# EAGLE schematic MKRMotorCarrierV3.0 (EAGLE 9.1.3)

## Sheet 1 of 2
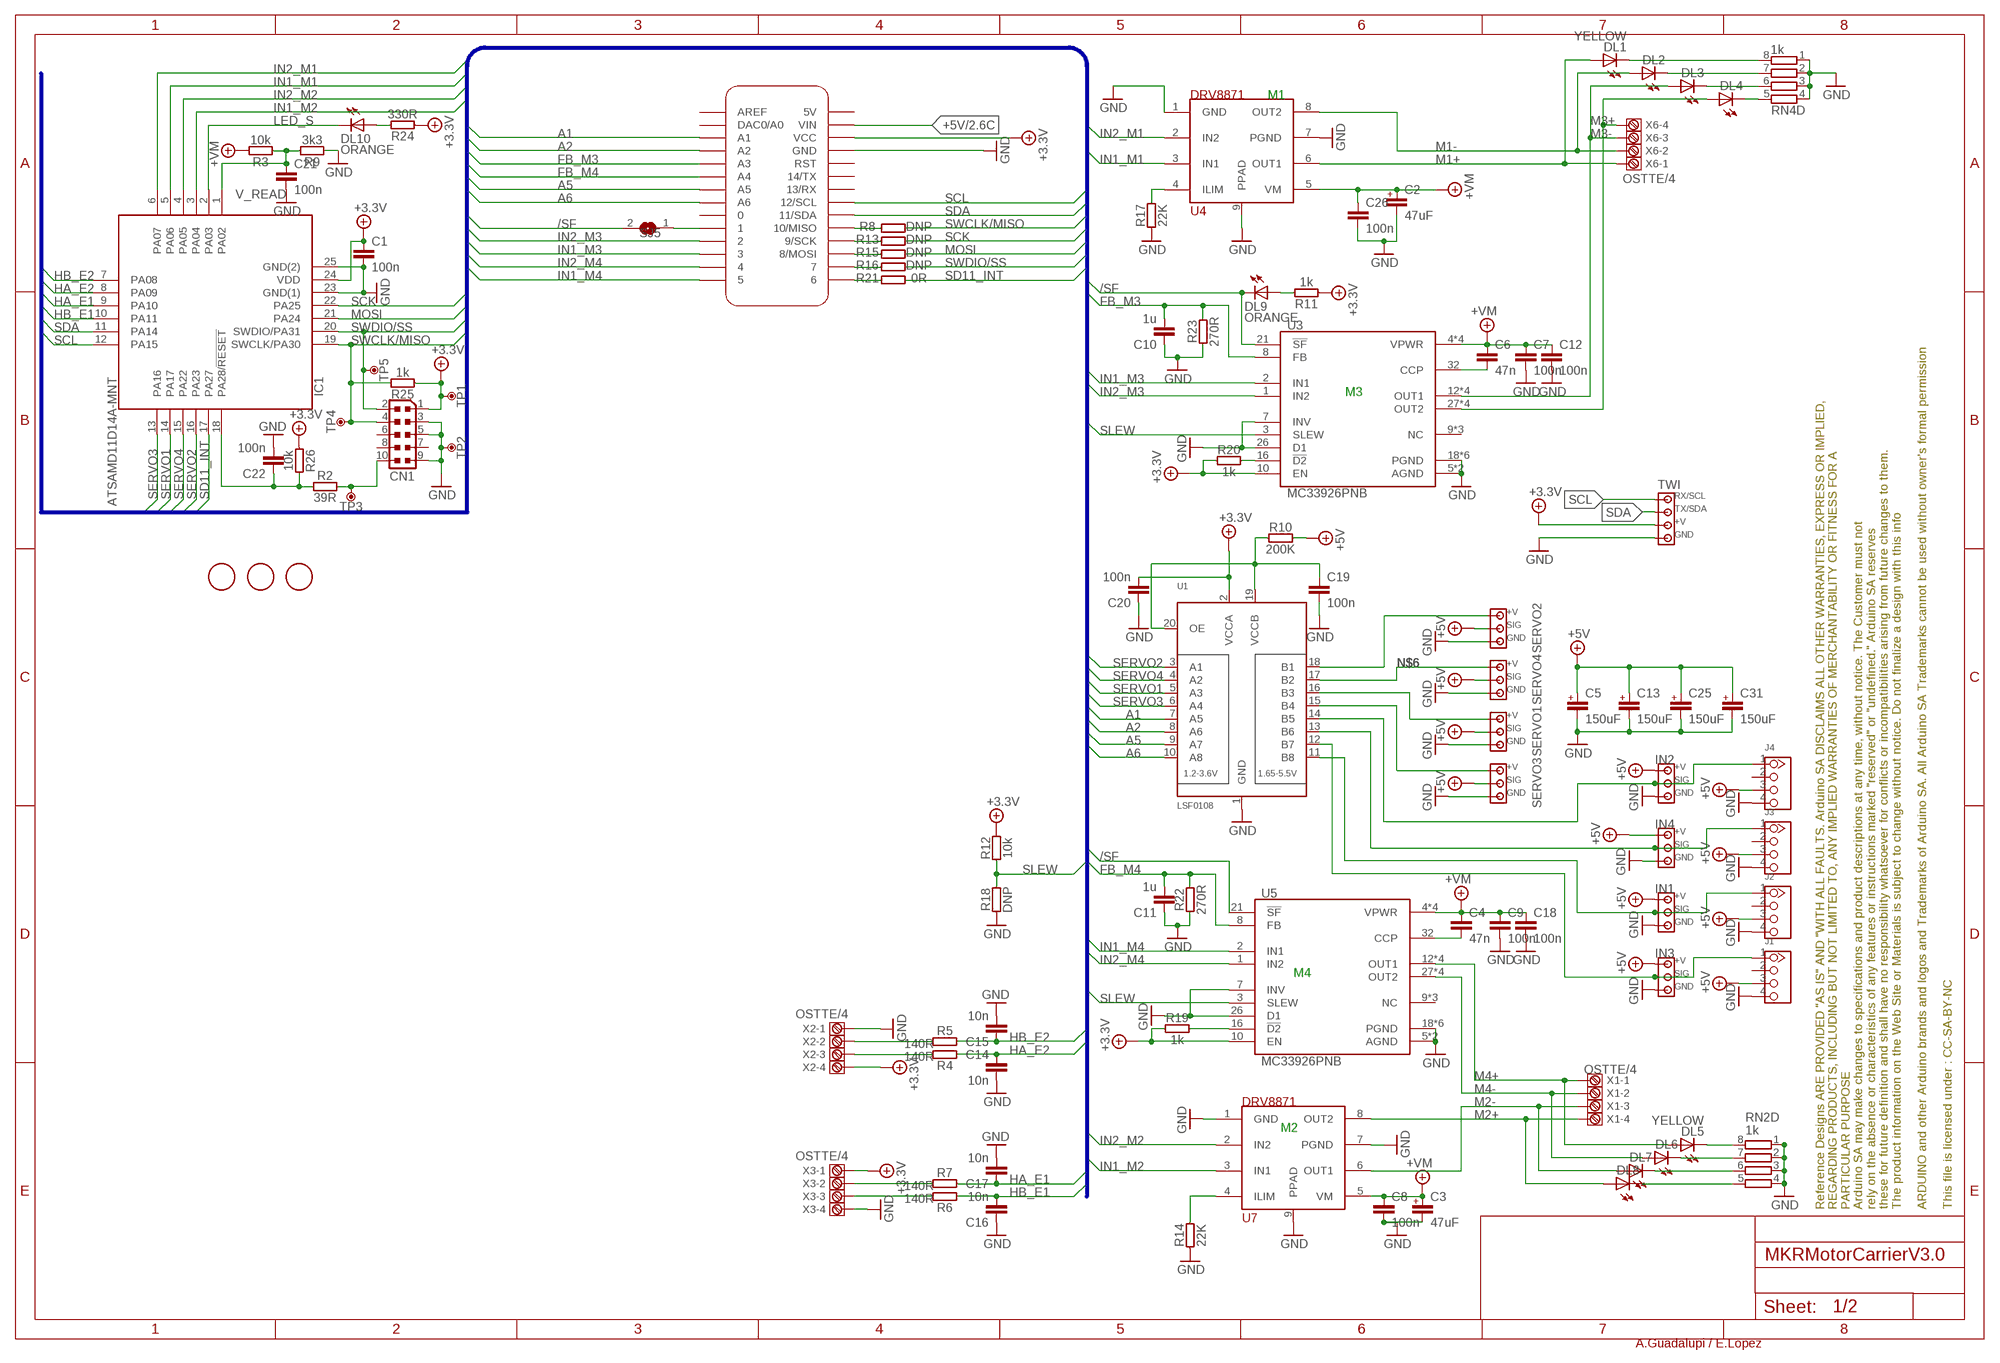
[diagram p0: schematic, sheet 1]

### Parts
C1  100n  C-100NF-0402  [0402-1005X55N]
C2  47uF  C+-47UFAVX-TCJ  [SMC_B]
C3  47uF  C+-47UFAVX-TCJ  [SMC_B]
C4  47n  C-47N-0402  [0402-1005X55N]
C5  150uF  C+PAN-C  [PANASONIC_C]
C6  47n  C-47N-0402  [0402-1005X55N]
C7  100n  C-100NF-0402  [0402-1005X55N]
C8  100n  C-100NF-0402  [0402-1005X55N]
C9  100n  C-100NF-0402  [0402-1005X55N]
C10  1u  C-1UF-0402  [0402-1005X55N]
C11  1u  C-1UF-0402  [0402-1005X55N]
C12  100n  C-100NF-0402  [0402-1005X55N]
C13  150uF  C+PAN-C  [PANASONIC_C]
C14  10n  C-10NF-0402  [0402-1005X55N]
C15  10n  C-10NF-0402  [0402-1005X55N]
C16  10n  C-10NF-0402  [0402-1005X55N]
C17  10n  C-10NF-0402  [0402-1005X55N]
C18  100n  C-100NF-0402  [0402-1005X55N]
C19  100n  C-100NF-0402  [0402-1005X55N]
C20  100n  C-100NF-0402  [0402-1005X55N]
C21  100n  C-100NF-0402  [0402-1005X55N]
C22  100n  C-100NF-0402  [0402-1005X55N]
C25  150uF  C+PAN-C  [PANASONIC_C]
C26  100n  C-100NF-0402  [0402-1005X55N]
C31  150uF  C+PAN-C  [PANASONIC_C]
CN1  DNP  JTAG_CONNECTOR-ROUND  [PINHEAD_2X05_127]
DL1  YELLOW  LED-YELLOW-0603  [LEDC1608X80N-AK]
DL2  YELLOW  LED-YELLOW-0603  [LEDC1608X80N-AK]
DL3  YELLOW  LED-YELLOW-0603  [LEDC1608X80N-AK]
DL4  YELLOW  LED-YELLOW-0603  [LEDC1608X80N-AK]
DL5  YELLOW  LED-YELLOW-0603  [LEDC1608X80N-AK]
DL6  YELLOW  LED-YELLOW-0603  [LEDC1608X80N-AK]
DL7  YELLOW  LED-YELLOW-0603  [LEDC1608X80N-AK]
DL8  YELLOW  LED-YELLOW-0603  [LEDC1608X80N-AK]
DL9  ORANGE  LED-ORANGE-0603  [LEDC1608X80N-AK]
DL10  ORANGE  LED-ORANGE-0603  [LEDC1608X80N-AK]
FRAME2  DNP  A3-FRAME-STANDARD  [FRAME]
IC1  ATSAMD11D14A-MNT  [QFN50P400X400X90-25N]
IN1  DNP  MODULINO-3-DNPSM  [MODULINO-3SM]
IN2  DNP  MODULINO-3-DNPSM  [MODULINO-3SM]
IN3  DNP  MODULINO-3-DNPSM  [MODULINO-3SM]
IN4  DNP  MODULINO-3-DNPSM  [MODULINO-3SM]
J1  DNP  GROVE-CONNECTOR-DNP  [HW4-2.0]
J2  DNP  GROVE-CONNECTOR-DNP  [HW4-2.0]
J3  DNP  GROVE-CONNECTOR-DNP  [HW4-2.0]
J4  DNP  GROVE-CONNECTOR-DNP  [HW4-2.0]
R2  39R  R-39R-0402  [0402-1005X55N]
R3  10k  R-10K-0402  [0402-1005X55N]
R4  140R  R-140R-0402  [0402-1005X55N]
R5  140R  R-140R-0402  [0402-1005X55N]
R6  140R  R-140R-0402  [0402-1005X55N]
R7  140R  R-140R-0402  [0402-1005X55N]
R8  DNP  R-DNP-0402  [0402-1005X55N]
R9  3k3  R-3K3-0402  [0402-1005X55N]
R10  200K  R-200K-0402  [0402-1005X55N]
R11  1k  R-1K-0402  [0402-1005X55N]
R12  10k  R-10K-0402  [0402-1005X55N]
R13  DNP  R-DNP-0402  [0402-1005X55N]
R14  22K  R-22K-0402  [0402-1005X55N]
R15  DNP  R-DNP-0402  [0402-1005X55N]
R16  DNP  R-DNP-0402  [0402-1005X55N]
R17  22K  R-22K-0402  [0402-1005X55N]
R18  DNP  R-DNP-0402  [0402-1005X55N]
R19  1k  R-1K-0402  [0402-1005X55N]
R20  1k  R-1K-0402  [0402-1005X55N]
R21  0R  R-0R-0402  [0402-1005X55N]
R22  270R  R-270R-0402  [0402-1005X55N]
R23  270R  R-270R-0402  [0402-1005X55N]
R24  330R  R-330R-0402  [0402-1005X55N]
R25  1k  R-1K-0402  [0402-1005X55N]
R26  10k  R-10K-0402  [0402-1005X55N]
RN2  1k  4R-N-1KCAY16  [CAY16]
RN4  1k  4R-N-1KCAY16  [CAY16]
SERVO1  DNP  MODULINO-3-DNPSM  [MODULINO-3SM]
SERVO2  DNP  MODULINO-3-DNPSM  [MODULINO-3SM]
SERVO3  DNP  MODULINO-3-DNPSM  [MODULINO-3SM]
SERVO4  DNP  MODULINO-3-DNPSM  [MODULINO-3SM]
SJ5  SJ  [SJ]
TP1  DNP  TPTP-1.00MM  [TP-1.00MM]
TP2  DNP  TPTP-1.00MM  [TP-1.00MM]
TP3  DNP  TPTP-1.00MM  [TP-1.00MM]
TP4  DNP  TPTP-1.00MM  [TP-1.00MM]
TP5  DNP  TPTP-1.00MM  [TP-1.00MM]
TWI  -  MODULINO-4  [MODULINO-4]
U1  LSF0108  LSF0108PWR  [TSSOP20]
U3  MC33926PNB  [32-PQFN(8X8)]
U4  DRV8871  [SOIC127P600X170-8N]
U5  MC33926PNB  [32-PQFN(8X8)]
U7  DRV8871  [SOIC127P600X170-8N]
U$1  MKRBOARD4CARRIER  [MKRBOARD-4CARRIER]
U$33  DNP  FIDUCIAL-1.5MM  [FD-1-1.5]
U$34  DNP  FIDUCIAL-1.5MM  [FD-1-1.5]
U$35  DNP  FIDUCIAL-1.5MM  [FD-1-1.5]
X1  OSTTE/4  [OSTTE/4]
X2  OSTTE/4  [OSTTE/4]
X3  OSTTE/4  [OSTTE/4]
X6  OSTTE/4  [OSTTE/4]

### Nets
+3.3V: C1.1 C20.2 CN1.1 IC1.24(VDD) R11.1 R12.2 R19.1 R20.1 R24.1 R25.1 R26.1 TP1.X TWI.3 U1.2(VCCA) U3.10(EN) U5.10(EN) U$1.VCC X2.4 X3.1 ; also sheet 2
+5V: C5.+ C13.+ C25.+ C31.+ IN1.1 IN2.1 IN3.1 IN4.1 J1.3 J2.3 J3.3 J4.3 R10.2 SERVO1.2 SERVO2.2 SERVO3.2 SERVO4.2 U$1.VIN ; also sheet 2
+VM: C2.+ C3.+ C4.1 C6.1 C7.1 C8.1 C9.1 C12.1 C18.1 C26.1 R3.2 U3.4(VPWR) U3.6(VPWR) U3.11(VPWR) U3.31(VPWR) U4.5(VM) U5.4(VPWR) U5.6(VPWR) U5.11(VPWR) U5.31(VPWR) U7.5(VM) ; also sheet 2
/SF: DL9.C SJ5.2 U3.21(!SF) U5.21(!SF)
A1: U1.7(A5) U$1.A1
A2: U1.8(A6) U$1.A2
A5: U1.9(A7) U$1.A5
A6: U1.10(A8) U$1.A6
FB_M3: C10.2 R23.2 U3.8(FB) U$1.A3
FB_M4: C11.2 R22.2 U5.8(FB) U$1.A4
GND: C1.2 C2.- C3.- C5.- C7.2 C8.2 C9.2 C10.1 C11.1 C12.2 C13.- C14.1 C15.2 C16.1 C17.2 C18.2 C19.2 C20.1 C21.2 C22.2 C25.- C26.2 C31.- CN1.3 CN1.5 CN1.9 IC1.23(GND(1)) IC1.25(GND(2)) IN1.3 IN2.3 IN3.3 IN4.3 J1.4 J2.4 J3.4 J4.4 R9.1 R14.1 R17.1 R18.1 R22.1 R23.1 RN2.1 RN2.2 RN2.3 RN2.4 RN4.1 RN4.2 RN4.3 RN4.4 SERVO1.3 SERVO2.3 SERVO3.3 SERVO4.3 TP2.X TWI.4 U1.1(GND) U3.5(AGND) U3.7(INV) U3.18(PGND) U3.19(PGND) U3.20(PGND) U3.22(PGND) U3.23(PGND) U3.24(PGND) U3.26(D1) U3.EPAD(AGND) U4.1(GND) U4.7(PGND) U4.9(PPAD) U5.5(AGND) U5.7(INV) U5.18(PGND) U5.19(PGND) U5.20(PGND) U5.22(PGND) U5.23(PGND) U5.24(PGND) U5.26(D1) U5.EPAD(AGND) U7.1(GND) U7.7(PGND) U7.9(PPAD) U$1.GND X2.1 X3.4 ; also sheet 2
HA_E1: C17.1 IC1.9(PA10) R7.1
HA_E2: C14.2 IC1.8(PA09) R4.1
HB_E1: C16.2 IC1.10(PA11) R6.1
HB_E2: C15.1 IC1.7(PA08) R5.1
IN1_A6: IN1.2 J2.1 U1.11(B8)
IN1_M1: IC1.5(PA06) U4.3(IN1)
IN1_M2: IC1.3(PA04) U7.3(IN1)
IN1_M3: U3.2(IN1) U$1.3
IN1_M4: U5.2(IN1) U$1.5
IN2_A1: IN2.2 J4.1 U1.14(B5)
IN2_M1: IC1.6(PA07) U4.2(IN2)
IN2_M2: IC1.4(PA05) U7.2(IN2)
IN2_M3: U3.1(IN2) U$1.2
IN2_M4: U5.1(IN2) U$1.4
IN3_A5: IN3.2 J1.1 U1.12(B7)
IN4_A2: IN4.2 J3.1 U1.13(B6)
LED_S: DL10.C IC1.2(PA03)
M1+: DL1.A U4.6(OUT1) X6.1
M1-: DL2.A U4.8(OUT2) X6.2
M2+: DL8.A U7.8(OUT2) X1.4
M2-: DL7.A U7.6(OUT1) X1.3
M3+: DL4.A U3.27(OUT2) U3.28(OUT2) U3.29(OUT2) U3.30(OUT2) X6.4
M3-: DL3.A U3.12(OUT1) U3.13(OUT1) U3.14(OUT1) U3.15(OUT1) X6.3
M4+: DL5.A U5.12(OUT1) U5.13(OUT1) U5.14(OUT1) U5.15(OUT1) X1.1
M4-: DL6.A U5.27(OUT2) U5.28(OUT2) U5.29(OUT2) U5.30(OUT2) X1.2
MOSI: IC1.21(PA24) R15.1
N$2: R6.2 X3.3
N$4: SERVO1.1 U1.16(B3)
N$6: SERVO4.1 U1.17(B2)
N$7: SERVO2.1 U1.18(B1)
N$9: SERVO3.1 U1.15(B4)
N$10: R7.2 X3.2
N$11: R5.2 X2.2
N$12: R4.2 X2.3
N$13: DL9.A R11.2
N$14: CN1.10 R2.2 TP3.X
N$15: C22.1 IC1.18(PA28/!RESET) R2.1 R26.2
N$16: SJ5.1 U$1.1
N$17: DL1.C RN4.8
N$18: C19.1 R10.1 U1.19(VCCB) U1.20(OE)
N$20: DL2.C RN4.7
N$21: DL3.C RN4.6
N$24: DL5.C RN2.8
N$25: DL4.C RN4.5
N$26: DL6.C RN2.7
N$28: C6.2 U3.32(CCP)
N$30: C4.2 U5.32(CCP)
N$31: DL7.C RN2.6
N$32: DL8.C RN2.5
N$35: R20.2 U3.16(!D2)
N$36: R17.2 U4.4(ILIM)
N$37: R19.2 U5.16(!D2)
N$38: R21.1 U$1.6
N$39: R14.2 U7.4(ILIM)
N$40: R8.2 U$1.10(10/MISO)
N$41: R13.2 U$1.9(9/SCK)
N$42: DL10.A R24.2
N$43: R15.2 U$1.8(8/MOSI)
N$45: R16.2 U$1.7
SCK: IC1.22(PA25) R13.1
SCL: IC1.12(PA15) TWI.1 U$1.12(12/SCL)
SD11_INT: IC1.17(PA27) R21.2
SDA: IC1.11(PA14) TWI.2 U$1.11(11/SDA)
SERVO1: IC1.14(PA17) U1.5(A3)
SERVO2: IC1.16(PA23) U1.3(A1)
SERVO3: IC1.13(PA16) U1.6(A4)
SERVO4: IC1.15(PA22) U1.4(A2)
SLEW: R12.1 R18.2 U3.3(SLEW) U5.3(SLEW)
SWCLK/MISO: CN1.4 IC1.19(SWCLK/PA30) R8.1 R25.2 TP4.X
SWDIO/SS: CN1.2 IC1.20(SWDIO/PA31) R16.1 TP5.X
V_READ: C21.1 IC1.1(PA02) R3.1 R9.2
Unconnected: CN1.6 CN1.7 CN1.8 J1.2 J2.2 J3.2 J4.2 U3.9(NC) U3.17(NC) U3.25(NC) U5.9(NC) U5.17(NC) U5.25(NC) U$1.0 U$1.5V U$1.13(13/RX) U$1.14(14/TX) U$1.A0(DAC0/A0) U$1.AREF U$1.RST

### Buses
MOSI,MISO,SCK,SS,SDA,SCL,A1,A2,A4,A3,A6,A5,FB_M3,FB_M4,IN1_M3,IN1_M4,IN1_M1,IN1_M2,IN2_M1,IN2_M2,IN2_M3,IN2_M4,SERVO1,SERVO2,SERVO3,SERVO4,HA_E1,HA_E2,HB_E1,HB_E2,VIN,/SF,SLEW,SD11_INT,SWDIO/SS,SWCLK/MISO

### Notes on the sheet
- M1
- M3
- M4
- M2
- A.Guadalupi / E.Lopez

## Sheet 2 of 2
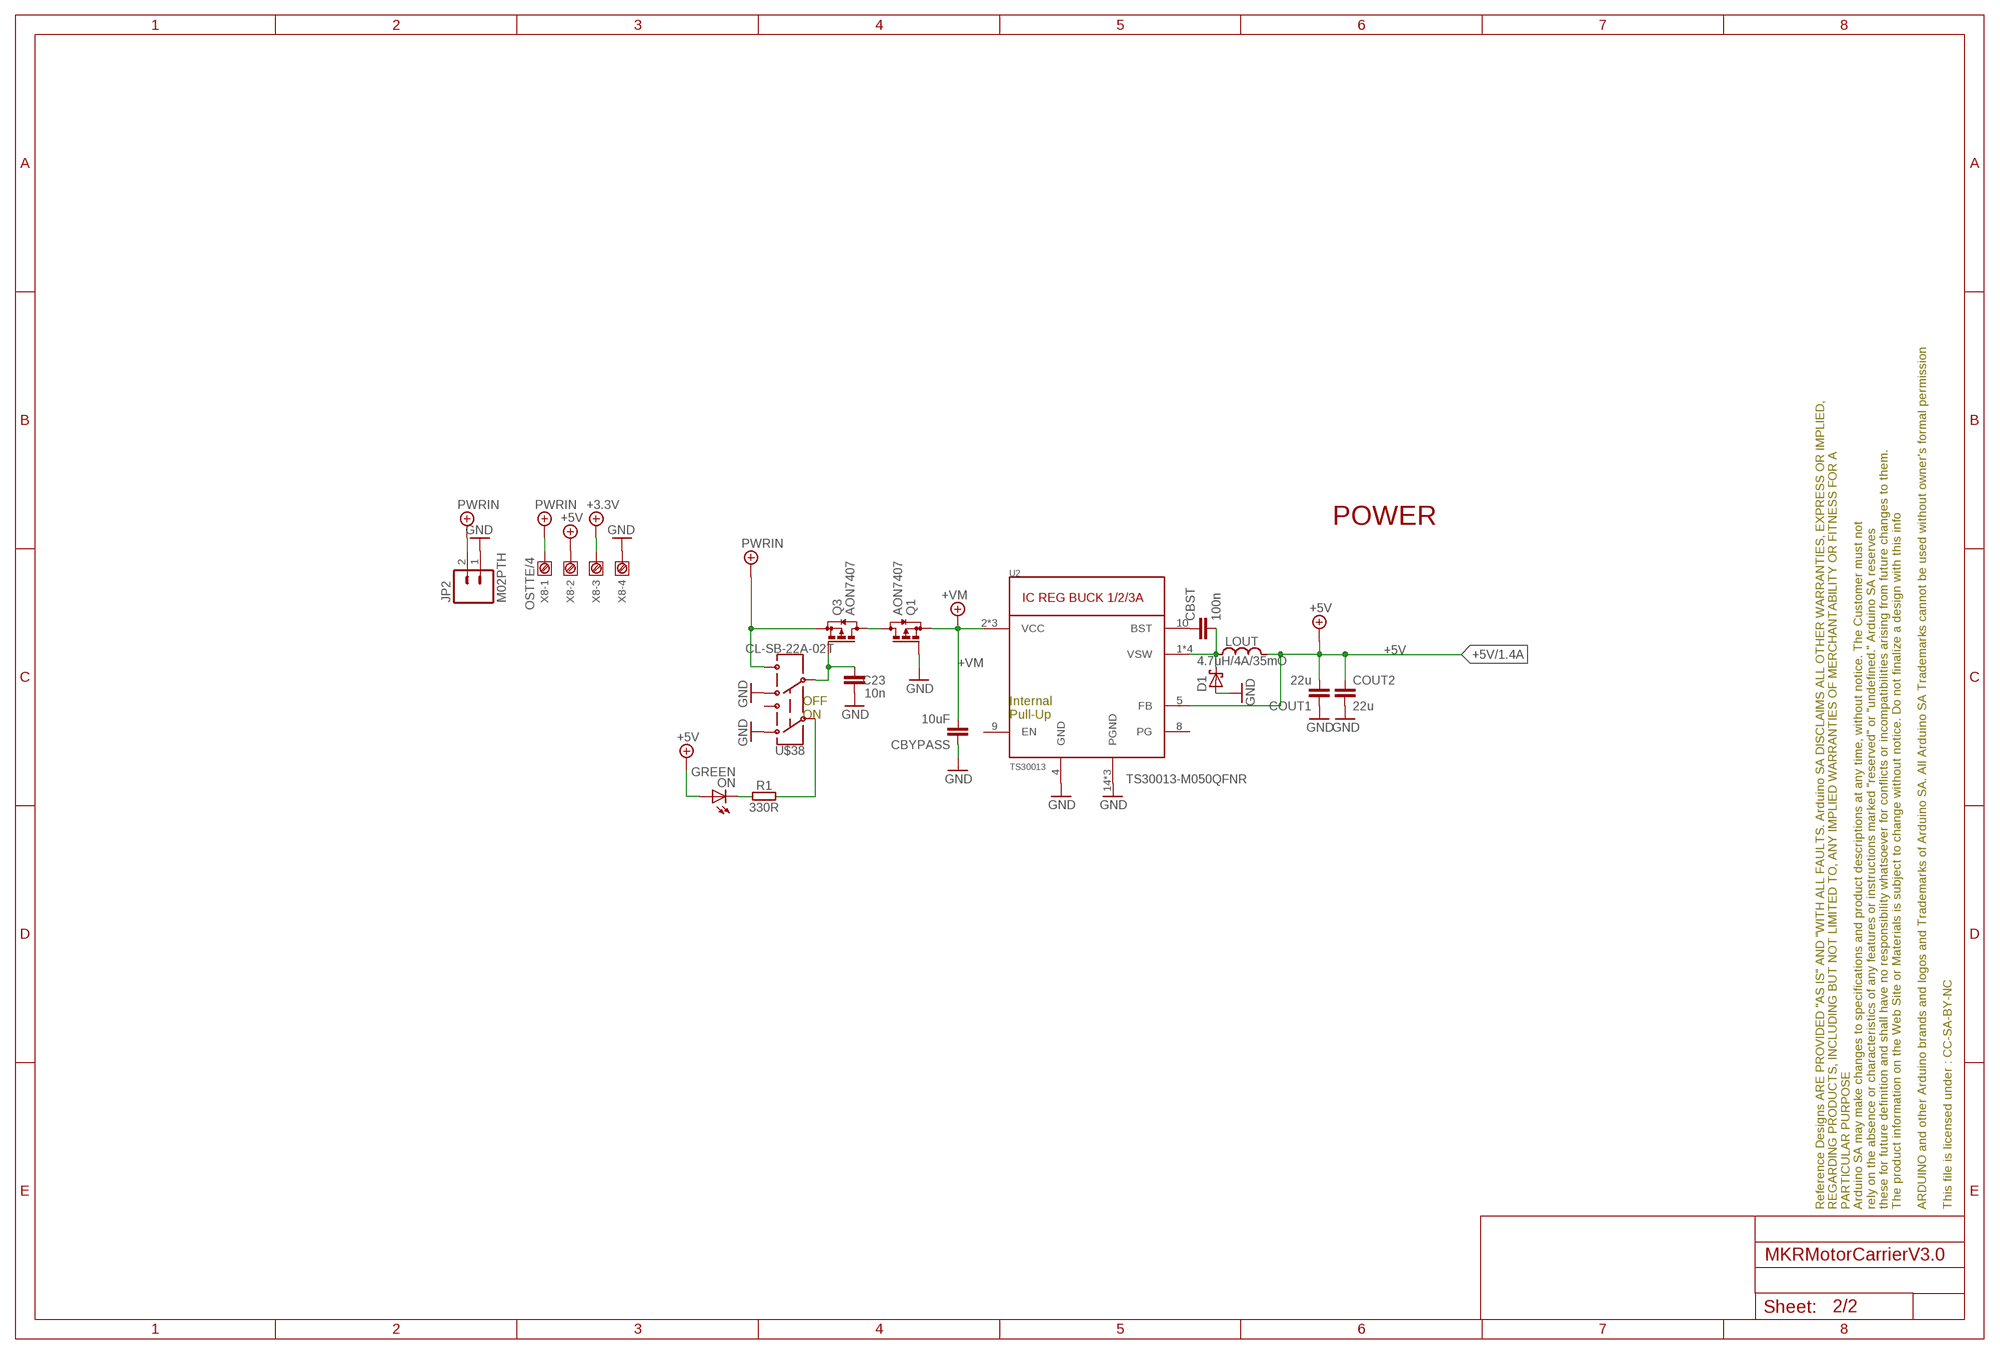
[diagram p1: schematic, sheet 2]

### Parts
C23  10n  C-10NF-0402  [0402-1005X55N]
CBST  100n  C-100NF-0402  [0402-1005X55N]
CBYPASS  10uF  C-10UF-1206  [C1206]
COUT1  22u  C-22U-0805  [0805-R2013X50N]
COUT2  22u  C-22U-0805  [0805-R2013X50N]
D1  40V/5A  D_SCHOTTKY-PMEG4050EP  [SOD-128]
FRAME1  DNP  A3-FRAME-NO-BAN  [FRAME-NO-BAN]
JP2  M02PTH  [1X02]
LOUT  4.7uH/4A/35mO  LVLS6045EX-4R7M  [6X6_NON-STANDARD]
ON  GREEN  LED-GREEN-0603  [LEDC1608X80N-AK]
Q1  AON7407  [DFN3X3_8L]
Q3  AON7407  [DFN3X3_8L]
R1  330R  R-330R-0402  [0402-1005X55N]
U2  TS30013  TS3001XTS30013  [QFN16]
U$38  CL-SB-22A-02T  [CL-SB-22A]
X8  OSTTE/4  [OSTTE/4]

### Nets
+3.3V: X8.3 ; also sheet 1
+5V: COUT1.2 COUT2.1 LOUT.P$2 ON.A U2.5(FB) X8.2 ; also sheet 1
+VM: CBYPASS.2 Q1.P$1(S) Q1.P$2(S) Q1.P$3(S) U2.2(VCC) U2.3(VCC) U2.11(VCC) ; also sheet 1
GND: C23.1 CBYPASS.1 COUT1.1 COUT2.2 D1.P$2(A) JP2.1 Q1.P$4(G) U2.4(GND) U2.14(PGND) U2.15(PGND) U2.17(PGND) U$38.P$1 U$38.P$4 X8.4 ; also sheet 1
N$3: CBST.1 U2.10(BST)
N$5: CBST.2 D1.P$1(C) LOUT.P$1 U2.1(VSW) U2.12(VSW) U2.13(VSW) U2.16(VSW)
N$19: R1.2 U$38.P$2
N$22: Q1.P$5(D) Q1.P$6(D) Q1.P$7(D) Q3.P$5(D) Q3.P$6(D) Q3.P$7(D)
N$23: C23.2 Q3.P$4(G) U$38.P$5
N$133: ON.C R1.1
PWRIN: JP2.2 Q3.P$1(S) Q3.P$2(S) Q3.P$3(S) U$38.P$6 X8.1
Unconnected: U2.8(PG) U2.9(EN) U$38.P$3

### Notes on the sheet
- POWER
- OFF
  ON
- Internal
  Pull-Up
- TS30013-M050QFNR

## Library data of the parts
C1 C7-C9 C12 C18-C22 C26 CBST = Arduino-rcl:C: SMD Capacitor; CODE-BCE: -; CODE-BCMI: -; CODE-TK2: -; DATASHEET: http://www.tdk.com/pdf/TDKMLCCCapRange.pdf; DISTRIBUTOR-LINK: http://www.digikey.com/product-detail/en/tdk-corporation/C1005X5R1H104K050BB/445-5942-1-ND/2443982; DISTRIBUTOR-PN: 445-5942-1-ND; MANUFACTURER: TDK; MANUFACTURER-PN: C1005X5R1H104K050BB
C2 C3 = BCMI-rcl:C+: TCJB106M025R0090: 10µF ±20% Molded Tantalum Polymer Capacitor 25V 1411 (3528 Metric) 90 mOhm; DATASHEET: http://catalogs.avx.com/TantalumNiobium.pdf; DISTRIBUTOR-LINK: https://www.digikey.se/products/en?keywords=%09478-9595-1-ND; DISTRIBUTOR-PN: 478-9595-1-ND; MANUFACTURER: AVX; MANUFACTURER-PN: TCNT476M016R0200A
C4 C6 = Arduino-rcl:C: SMD Capacitor; CODE-BCE: -; CODE-BCMI: -; CODE-TK2: -; DATASHEET: http://www.murata.com/~/media/webrenewal/support/library/catalog/products/capacitor/mlcc/c02e.pdf; DISTRIBUTOR-LINK: https://www.digikey.com/product-detail/en/murata-electronics-north-america/GRM155R71E473KA88D/490-3254-1-ND/702795; DISTRIBUTOR-PN: 490-3254-1-ND; MANUFACTURER: Murata; MANUFACTURER-PN: GRM155R71E473KA88D
C5 C13 C25 C31 = Arduino-rcl:C+: Polarized Capacitor; DATASHEET: https://industrial.panasonic.com/cdbs/www-data/pdf/RDE0000/DME0000COL92.pdf; DISTRIBUTOR-LINK: https://www.digikey.se/products/en?keywords=P15082CT-ND; DISTRIBUTOR-PN: P15082CT-ND; MANUFACTURER: Panasonic; MANUFACTURER-PN: EEE-FT1A151AR
C10 C11 = Arduino-rcl:C: SMD Capacitor; CODE-BCE: -; CODE-BCMI: -; CODE-TK2: -; DATASHEET: http://search.murata.co.jp/Ceramy/image/img/A01X/partnumbering_e_01.pdf; DISTRIBUTOR-LINK: http://www.digikey.com/product-detail/en/murata-electronics-north-america/GRM155R61E105KA12D/490-10017-1-ND/5026367; DISTRIBUTOR-PN: 490-10017-1-ND; MANUFACTURER: Murata; MANUFACTURER-PN: GRM155R61E105KA12D
C14-C17 C23 = Arduino-rcl:C: SMD Capacitor; CODE-BCE: -; CODE-BCMI: -; CODE-TK2: -; DATASHEET: http://search.murata.co.jp/Ceramy/image/img/A01X/partnumbering_e_01.pdf; DISTRIBUTOR-LINK: http://www.digikey.com/product-detail/en/murata-electronics-north-america/GRM155R71H103KA88J/490-6351-1-ND/3845548; DISTRIBUTOR-PN: 490-6351-1-ND; MANUFACTURER: Murata; MANUFACTURER-PN: GRM155R71H103KA88J
CBYPASS = Arduino-rcl:C: SMD Capacitor; CODE-BCE: -; CODE-BCMI: -; CODE-TK2: -; DATASHEET: https://product.tdk.com/en/products/common/pdf/mlcc_partnumber_description.pdf; DISTRIBUTOR-LINK: https://www.digikey.se/products/en?keywords=445-14694-1-ND; DISTRIBUTOR-PN: 445-14694-1-ND; MANUFACTURER: TDK Corporation; MANUFACTURER-PN: C3216X5R1V106K160AB
CN1 = Arduino-connectors:JTAG_CONNECTOR: 2x5 PASSO 1,27; CODE-BCE: DNP; CODE-TK2: DNP; DATASHEET: DNP; DISTRIBUTOR-LINK: DNP; DISTRIBUTOR-PN: DNP; MANUFACTURER: DNP; MANUFACTURER-PN: DNP
COUT1 COUT2 = BCMI-rcl:C: SMD Capacitor; DATASHEET: https://media.digikey.com/pdf/Data%20Sheets/Samsung%20PDFs/CL21A226MQCLQNC_character.pdf; DISTRIBUTOR-LINK: https://www.digikey.com/product-detail/en/samsung-electro-mechanics-america-inc/CL21A226MQCLQNC/1276-2412-1-ND/3890498; DISTRIBUTOR-PN: 1276-2412-1-ND; MANUFACTURER: Samsung; MANUFACTURER-PN: CL21A226MQCLQNC
D1 = Arduino-diodes:D_SCHOTTKY: Schottky Diodes; DATASHEET: https://assets.nexperia.com/documents/data-sheet/PMEG4050EP.pdf; DISTRIBUTOR-LINK: https://www.digikey.se/products/en?keywords=1727-5842-1-ND; DISTRIBUTOR-PN: 1727-5842-1-ND; MANUFACTURER: Nexperia USA Inc.; MANUFACTURER-PN: PMEG4050EP,115
DL1-DL8 = Arduino-diodes:LED: LED; DATASHEET: http://media.digikey.com/pdf/Data%20Sheets/Avago%20PDFs/HSMz-Czzz.pdf; DISTRIBUTOR-LINK: http://www.digikey.com/product-detail/en/broadcom-limited/HSMY-C190/516-1424-1-ND/637748; DISTRIBUTOR-PN: 516-1424-1-ND; MANUFACTURER: Avago; MANUFACTURER-PN: HSMY-C190
DL9 DL10 = Arduino-diodes:LED: LED; DATASHEET: http://media.digikey.com/pdf/Data%20Sheets/Avago%20PDFs/HSMz-Czzz.pdf; DISTRIBUTOR-LINK: http://www.digikey.com/product-detail/en/broadcom-limited/HSMD-C190/516-2489-1-ND/2744915; DISTRIBUTOR-PN: 516-2489-1-ND; MANUFACTURER: Avago; MANUFACTURER-PN: HSMD-C190
FRAME1 FRAME2 = Arduino-utility:A3-FRAME: Schematic frame; CODE-ARDUINO: DNP; DATASHEET: DNP; DISTRIBUTOR-LINK: DNP; DISTRIBUTOR-PN: DNP; MANUFACTURER: DNP; MANUFACTURER-PN: DNP
IC1 = ATSAMD11D14A-MNT:ATSAMD11D14A-MNT: ARM Microcontrollers - MCU Cortex-M0+, 16KB FLASH,4KB SRAM, USB - 24 QFN,105C, GREEN,1.6-3.6V,48MHz,USB Source: Datasheet; DATASHEEET: http://ww1.microchip.com/downloads/en/DeviceDoc/Atmel-42363-SAM-D11_Datasheet.pdf; DESCRIPTION: ARM Microcontrollers - MCU Cortex-M0+, 16KB FLASH,4KB SRAM, USB - 24 QFN,105C, GREEN,1.6-3.6V,48MHz,USB; DISTRIBUTOR-LINK: https://www.digikey.se/products/en?keywords=ATSAMD11D14A-MUTCT-ND; DISTRIBUTOR-PN: ATSAMD11D14A-MUTCT-ND; MANUFACTURER: Microchip; MANUFACTURER-PN: ATSAMD11D14A-MNT
IN1-IN4 SERVO1-SERVO4 = Arduino-connectors:MODULINO-3: Modulino 4 connector; DATASHEET: DNP; DISTRIBUTOR-LINK: DNP; DISTRIBUTOR-PN: DNP; MANUFACTURER: DNP; MANUFACTURER-PN: DNP
J1-J4 = Arduino-connectors:GROVE-CONNECTOR: Grove connector; CODE-BCE: DNP; CODE-TK2: DNP; DATASHEET: DNP; DISTRIBUTOR-LINK: DNP; DISTRIBUTOR-PN: DNP; MANUFACTURER: DNP; MANUFACTURER-PN: DNP
JP2 = MyLibrary:M02: Standard 2-pin 0.1" header. Use with
LOUT = Arduino-rcl:L: Inductors; DATASHEET: https://product.tdk.com/info/en/catalog/datasheets/inductor_commercial_power_vls6045ex_en.pdf; DISTRIBUTOR-LINK: https://www.digikey.se/products/en?keywords=445-173055-1-ND; DISTRIBUTOR-PN: 445-173055-1-ND; MANUFACTURER: TDK Corporation; MANUFACTURER-PN: VLS6045EX-4R7M
ON = BCMI-diodes:LED: LED; DATASHEET: http://media.digikey.com/pdf/Data%20Sheets/Avago%20PDFs/HSMz-Czzz.pdf; DISTRIBUTOR-LINK: http://www.digikey.com/product-detail/en/broadcom-limited/HSMG-C190/516-1425-1-ND/637749; DISTRIBUTOR-PN: 516-1425-1-ND; MANUFACTURER: Avago; MANUFACTURER-PN: HSMG-C190
Q1 Q3 = BCMI-transistors:AON7407: MOSFET P-CH 20V 14.5A 8DFN P-Channel Mosfet LEGEND VDS: Voltage Drain-Source ID: Drain Current RDS(ON): Drain-Source On-State Resistance VGS(TH): Gate-Source Threshold Voltage CISS: Drain-Source Input Capacitance SOT-23 Name VDS ID RDS(ON) VGS(TH) CISS Package Order Number AON7407 20V 14.5A mOhm --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; DATASHEET: http://aosmd.com/res/data_sheets/AON7407.pdf; DISTRIBUTOR-LINK: https://www.digikey.se/products/en?keywords=785-1306-1-ND; DISTRIBUTOR-PN: 785-1306-1-ND; MANUFACTURER: Alpha&Omega; MANUFACTURER-PN: AON7407
R1 R24 = Arduino-rcl:R: SMD Resistor; CODE-BCE: -; CODE-BCMI: -; CODE-TK2: -; DATASHEET: www.yageo.com.tw/exep/pages/download/literatures/PYu-R_INT-thick_7.pdf; DISTRIBUTOR-LINK: http://www.digikey.com/product-detail/en/yageo/RC0402FR-07330RL/311-330LRCT-ND/729541; DISTRIBUTOR-PN: 311-330LRCT-ND; MANUFACTURER: Yageo; MANUFACTURER-PN: RC0402FR-07330RL
R2 = Arduino-rcl:R: SMD Resistor; CODE-BCE: -; CODE-BCMI: -; CODE-TK2: -; DATASHEET: www.yageo.com.tw/exep/pages/download/literatures/PYu-R_INT-thick_7.pdf; DISTRIBUTOR-LINK: http://www.digikey.com/product-detail/en/yageo/RC0402FR-0739RL/311-39.0LRCT-ND/729549; DISTRIBUTOR-PN: 311-39.0LRCT-ND; MANUFACTURER: Yageo; MANUFACTURER-PN: RC0402FR-0739RL
R3 R12 R26 = Arduino-rcl:R: SMD Resistor; CODE-BCE: -; CODE-BCMI: -; CODE-TK2: -; DATASHEET: www.yageo.com.tw/exep/pages/download/literatures/PYu-R_INT-thick_7.pdf; DISTRIBUTOR-LINK: http://www.digikey.com/product-detail/en/yageo/RC0402FR-0710KL/311-10.0KLRCT-ND/729470; DISTRIBUTOR-PN: 311-10.0KLRCT-ND; MANUFACTURER: Yageo; MANUFACTURER-PN: RC0402FR-0710KL
R4-R7 = BCMI-rcl:R: SMD Resistor; DATASHEET: www.yageo.com.tw/exep/pages/download/literatures/PYu-R_INT-thick_7.pdf; DISTRIBUTOR-LINK: https://www.digikey.se/products/en/resistors/chip-resistor-surface-mount/52?k=resistor&k=&pkeyword=resistor&pv7=2&FV=fffc000d%2C400ad%2C400004%2C1f140000%2Cffe00034%2Cc0001&mnonly=0&ColumnSort=0&page=1&stock=1&quantity=0&ptm=0&fid=0&pageSize=500; DISTRIBUTOR-PN: 311-140LRCT-ND; MANUFACTURER: Yageo; MANUFACTURER-PN: RC0402FR-07140RL
R8 R13 R15 R16 R18 = Arduino-rcl:R: SMD Resistor; CODE-BCE: -; CODE-BCMI: -; CODE-TK2: -; DATASHEET: DNP; DISTRIBUTOR-LINK: DNP; DISTRIBUTOR-PN: DNP; MANUFACTURER: DNP; MANUFACTURER-PN: DNP
R9 = Arduino-rcl:R: SMD Resistor; CODE-BCE: -; CODE-BCMI: -; CODE-TK2: -; DATASHEET: www.yageo.com.tw/exep/pages/download/literatures/PYu-R_INT-thick_7.pdf; DISTRIBUTOR-LINK: https://www.digikey.com/product-detail/en/yageo/RC0402FR-073K3L/311-3.30KLRCT-ND/729527; DISTRIBUTOR-PN: 311-3.30KLRCT-ND; MANUFACTURER: Yageo; MANUFACTURER-PN: RC0402FR-073K3L
R10 = BCMI-rcl:R: SMD Resistor; DATASHEET: http://www.yageo.com/NewPortal/yageodocoutput?fileName=/pdf/R-Chip/PYu-AC_51_RoHS_L_6.pdf; DISTRIBUTOR-LINK: https://www.digikey.se/product-detail/en/yageo/AC0402FR-07200KL/YAG3452CT-ND/6006301; DISTRIBUTOR-PN: YAG3452CT-ND; MANUFACTURER: Yageo; MANUFACTURER-PN: AC0402FR-07200KL
R11 R19 R20 R25 = Arduino-rcl:R: SMD Resistor; CODE-BCE: -; CODE-BCMI: -; CODE-TK2: -; DATASHEET: www.yageo.com.tw/exep/pages/download/literatures/PYu-R_INT-thick_7.pdf; DISTRIBUTOR-LINK: http://www.digikey.com/product-detail/en/yageo/RC0402FR-071KL/311-1.00KLRCT-ND/729460; DISTRIBUTOR-PN: 311-1.00KLRCT-ND; MANUFACTURER: Yageo; MANUFACTURER-PN: RC0402FR-071KL
R14 R17 = Arduino-rcl:R: SMD Resistor; CODE-BCE: -; CODE-BCMI: -; CODE-TK2: -; DATASHEET: http://www.yageo.com/NewPortal/yageodocoutput?fileName=/pdf/R-Chip/PYu-AC_51_RoHS_L_6.pdf; DISTRIBUTOR-LINK: https://www.digikey.se/products/en?keywords=%09YAG3532CT-ND; DISTRIBUTOR-PN: YAG3532CT-ND; MANUFACTURER: Yageo; MANUFACTURER-PN: AC0402JR-0722KL
R21 = Arduino-rcl:R: SMD Resistor; CODE-BCE: SP0039; CODE-BCMI: 0039; CODE-TK2: -; DATASHEET: www.yageo.com.tw/exep/pages/download/literatures/PYu-R_INT-thick_7.pdf; DISTRIBUTOR-LINK: http://www.digikey.com/product-detail/en/yageo/RC0402FR-070RL/311-0.0LRCT-ND/2827888; DISTRIBUTOR-PN: 311-0.0LRCT-ND; MANUFACTURER: Yageo; MANUFACTURER-PN: RC0402FR-070RL
R22 R23 = Arduino-rcl:R: SMD Resistor; CODE-BCE: -; CODE-BCMI: -; CODE-TK2: -; DATASHEET: www.yageo.com.tw/exep/pages/download/literatures/PYu-R_INT-thick_7.pdf; DISTRIBUTOR-LINK: http://www.digikey.com/product-detail/en/yageo/RC0402JR-07270RL/311-270JRCT-ND/729395; DISTRIBUTOR-PN: 311-270JRCT-ND; MANUFACTURER: Yageo; MANUFACTURER-PN: RC0402JR-07270RL
RN2 RN4 = Arduino-rcl:4R-N: Array Chip Resistor Source: RS Component / Phycomp; CODE-BCE: SP0005; CODE-BCMI: 0005; CODE-TK2: CAY16-102J4GLF; DATASHEET: http://www.bourns.com/docs/Product-Datasheets/CATCAY.pdf; DISTRIBUTOR-LINK: https://www.digikey.com/product-detail/en/bourns-inc/CAY16-102J4LF/CAY16-102J4LFCT-ND/3437828; DISTRIBUTOR-PN: CAY16-102J4LFCT-ND; MANUFACTURER: Bourns Inc.; MANUFACTURER-PN: CAY16-102J4LF
SJ5 = jumper:SJ: SMD solder JUMPER
TP1-TP5 = Arduino-utility:TP: Testpoint; DATASHEET: DNP; DISTRIBUTOR-LINK: DNP; DISTRIBUTOR-PN: DNP; MANUFACTURER: DNP; MANUFACTURER-PN: DNP
TWI = Arduino-connectors:MODULINO-4: Modulino 4 connector; CODE-BCE: -; CODE-TK2: -; DATASHEET: -; DISTRIBUTOR-LINK: -; DISTRIBUTOR-PN: -; MANUFACTURER: -; MANUFACTURER-PN: -
U1 = Arduino-ICs:LSF0108PWR: Voltage Level Translator Bidirectional 1 Circuit 8 Channel 100Mbps; CODE-BCE: -; CODE-TK2: -; DATASHEET: http://www.ti.com/lit/ds/symlink/lsf0108.pdf; DISTRIBUTOR-LINK: https://www.digikey.com/product-detail/en/texas-instruments/LSF0108PWR/296-37828-1-ND/4876357; DISTRIBUTOR-PN: 296-37828-1-ND; MANUFACTURER: Texas Instruments; MANUFACTURER-PN: LSF0108PWR
U2 = Arduino-ICs:TS3001X: TS30011/12/13 Buck Switching Regulator IC Positive Fixed/adjustable 5V 1 Output 1A/2A/3A 16-VFQFN Exposed Pad; DATASHEET: http://www.semtech.com/images/datasheet/ts30011_12_13.pdf; DISTRIBUTOR: Digikey; DISTRIBUTOR-LINK: https://www.digikey.se/products/en?keywords=TS30013-M050QFNRCT-ND; DISTRIBUTOR-PN: TS30013-M050QFNRCT-ND; MANUFACTURER: Semtech Corporation; MANUFACTURER-PN: TS30013-M050QFNR
U3 U5 = MC33926PNB-newSymbol:MC33926PNB: Motor / Motion / Ignition Controllers & Drivers THROTTLE CTRL H-BRIDGE Source: Datasheet; DATASHEET: https://www.nxp.com/docs/en/data-sheet/MC33926.pdf; DISTRIBUTOR-LINK: https://www.digikey.se/products/en?keywords=MC33926PNBR2CT-ND; DISTRIBUTOR-PN: MC33926PNBR2CT-ND; MANUFACTURER: NXP; MANUFACTURER-PN: MC33926PNBR2
U4 U7 = SOIC127P600X170-8N:DRV8871; DATASHEET: http://www.ti.com/lit/ds/symlink/drv8871.pdf; DESCRIPTION: Motor Driver 3.6A 6.5-45v; DISTRIBUTOR-LINK: https://www.digikey.se/products/en?keywords=296-43024-1-ND; DISTRIBUTOR-PN: 296-43024-1-ND; MANUFACTURER: Texas Instruments; MANUFACTURER-PN: DRV8871DDAR
U$1 = BCMI-utility:MKRBOARD
U$33-U$35 = Arduino-utility:FIDUCIAL: Fiducial mount; CODE-BCE: DNP; CODE-BCMI: DNP; CODE-TK2: DNP; DATASHEET: DNP; DISTRIBUTOR-LINK: DNP; DISTRIBUTOR-PN: DNP; MANUFACTURER: DNP; MANUFACTURER-PN: DNP
U$38 = BCMI-Switches:CL-SB-22A-02T: Slide Switch DPDT Surface Mount; DATASHEET: https://www.nidec-copal-electronics.com/e/catalog/switch/cl-sb.pdf; DISTRIBUTOR-LINK: https://www.digikey.se/products/en?keywords=563-1339-1-ND; DISTRIBUTOR-PN: 563-1339-1-ND; MANUFACTURER: Copal Electronics; MANUFACTURER-PN: CL-SB-22A-02T
X1-X3 X6 X8 = BCMI-connectors:OSTTE/4: TERM BLOCK 3.5MM VERT 4POS PCB 0.138" (3.50mm) Through Hole 10A 125V 16-26 AWG Blue Screw M2; DATASHEET: http://www.on-shore.com/wp-content/uploads/2015/09/osttexx0161.pdf; DISTRIBUTOR: Digikey; DISTRIBUTOR-LINK: https://www.digikey.se/product-detail/en/on-shore-technology-inc/OSTTE040161/ED2637-ND/614586; DISTRIBUTOR-PN: ED2637-ND; MANUFACTURER: On Shore Technologies; MANUFACTURER-PN: OSTTE040161

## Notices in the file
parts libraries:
Arduino-utility: Copyright (c) 2016-2017 Arduino LLC. All right reserved.
Arduino-utility: This file is licensed under : CC-SA-BY-NC
